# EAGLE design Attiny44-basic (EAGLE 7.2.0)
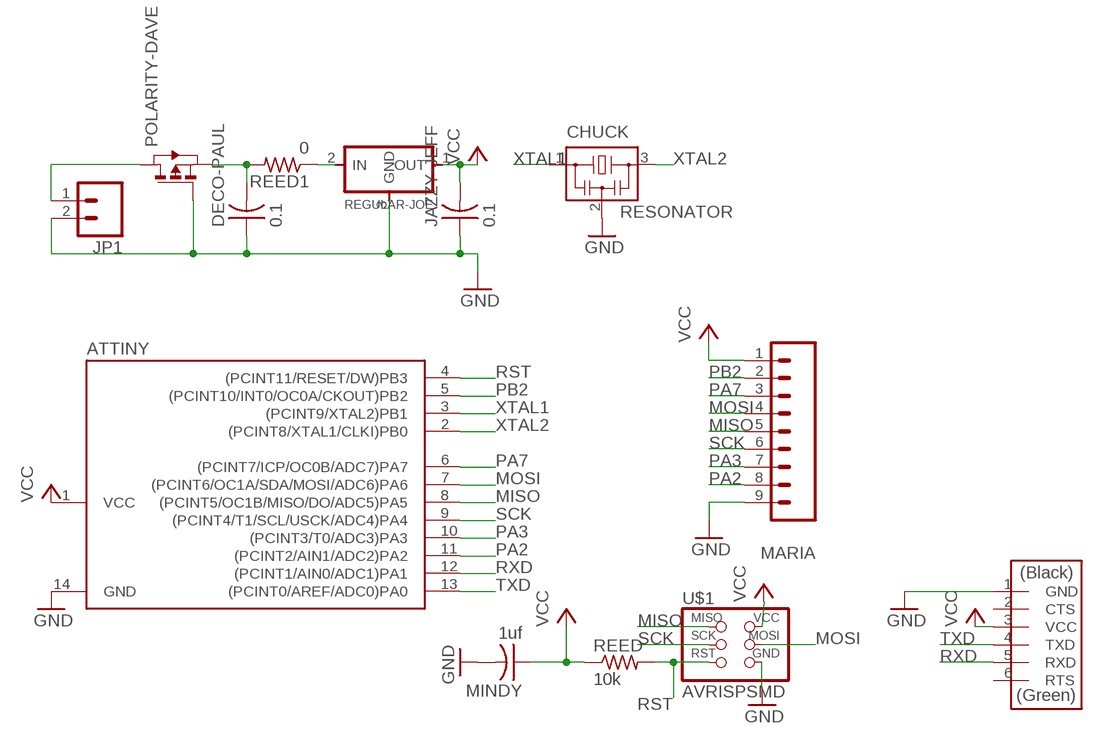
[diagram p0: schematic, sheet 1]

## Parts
ATTINY  ATTINY44-SSU  [SOIC14]
CHUCK  RESONATOR  [EFOBM]
DECO-PAUL  0.1  CAP-US1206  [C1206]
FTDINO  FTDI-SMD-HEADER  [1X06SMD]
JAZZY-JEFF  0.1  CAP-US1206  [C1206]
JP1  M02POLAR_LOCK  [MOLEX-1X2_LOCK]
MARIA  M09LONGPADS  [1X09_LONGPADS]
MINDY  1uf  CAP-US1206  [C1206]
POLARITY-DAVE  PMOSFETSOT23  [SOT-23]
REED  10k  RES-US1206  [R1206]
REED1  0  RES-US1206  [R1206]
REGULAR-JOE  REGULATORSOT23  [SOT23]
U$1  AVRISPSMD  [2X03SMD]

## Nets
GND: ATTINY.14(GND) CHUCK.2 DECO-PAUL.1 FTDINO.1(GND) JAZZY-JEFF.1 JP1.2 MARIA.9 MINDY.2 POLARITY-DAVE.3(G) REGULAR-JOE.3(GND) U$1.6(GND)
MISO: ATTINY.8((PCINT5/OC1B/MISO/DO/ADC5)PA5) MARIA.5 U$1.1(MISO)
MOSI: ATTINY.7((PCINT6/OC1A/SDA/MOSI/ADC6)PA6) MARIA.4 U$1.4(MOSI)
N$1: DECO-PAUL.2 POLARITY-DAVE.2(S) REED1.2
N$3: REED1.1 REGULAR-JOE.2(IN)
N$6: JP1.1 POLARITY-DAVE.1(D)
PA2: ATTINY.11((PCINT2/AIN1/ADC2)PA2) MARIA.8
PA3: ATTINY.10((PCINT3/T0/ADC3)PA3) MARIA.7
PA7: ATTINY.6((PCINT7/ICP/OC0B/ADC7)PA7) MARIA.3
PB2: ATTINY.5((PCINT10/INT0/OC0A/CKOUT)PB2) MARIA.2
RST: ATTINY.4((PCINT11/RESET/DW)PB3) REED.2 U$1.5(RST)
RXD: ATTINY.12((PCINT1/AIN0/ADC1)PA1) FTDINO.5(RXD)
SCK: ATTINY.9((PCINT4/T1/SCL/USCK/ADC4)PA4) MARIA.6 U$1.3(SCK)
TXD: ATTINY.13((PCINT0/AREF/ADC0)PA0) FTDINO.4(TXD)
VCC: ATTINY.1(VCC) FTDINO.3(VCC) JAZZY-JEFF.2 MARIA.1 MINDY.1 REED.1 REGULAR-JOE.1(OUT) U$1.2(VCC)
XTAL1: ATTINY.3((PCINT9/XTAL2)PB1) CHUCK.1
XTAL2: ATTINY.2((PCINT8/XTAL1/CLKI)PB0) CHUCK.3
Unconnected: FTDINO.2(CTS) FTDINO.6(RTS)

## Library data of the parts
ATTINY = 01fab:ATTINY44
CHUCK = 01fab:RESONATOR
DECO-PAUL JAZZY-JEFF MINDY = 01fab:CAP-US
FTDINO = 01fab:FTDI-SMD-HEADER
JP1 = 01_SparkFun:M02: Header 2
MARIA = 01_SparkFun:M09: Header 9 Standard 9-pin 0.1" header. Use with straight break away headers (SKU : PRT-00116), right angle break away headers (PRT-00553), swiss pins (PRT-00743), machine pins (PRT-00117), and female headers (PRT-00115).
POLARITY-DAVE = 01fab:PMOSFET: MOS FET
REED REED1 = 01fab:RES-US: Resistor (US Symbol)
REGULAR-JOE = 01fab:REGULATOR
U$1 = 01fab:AVRISP

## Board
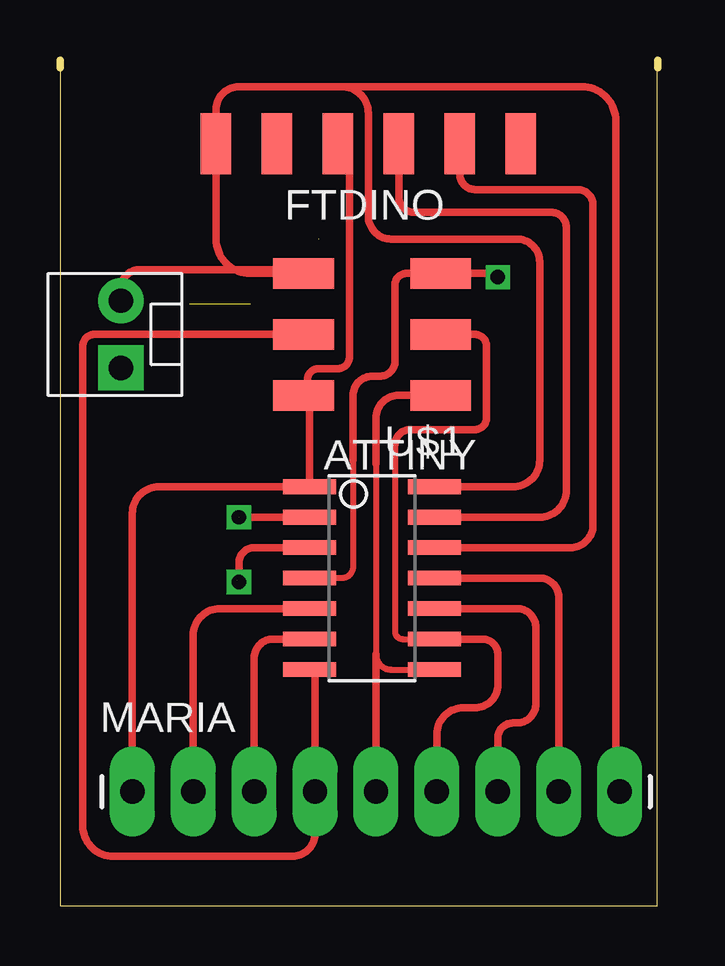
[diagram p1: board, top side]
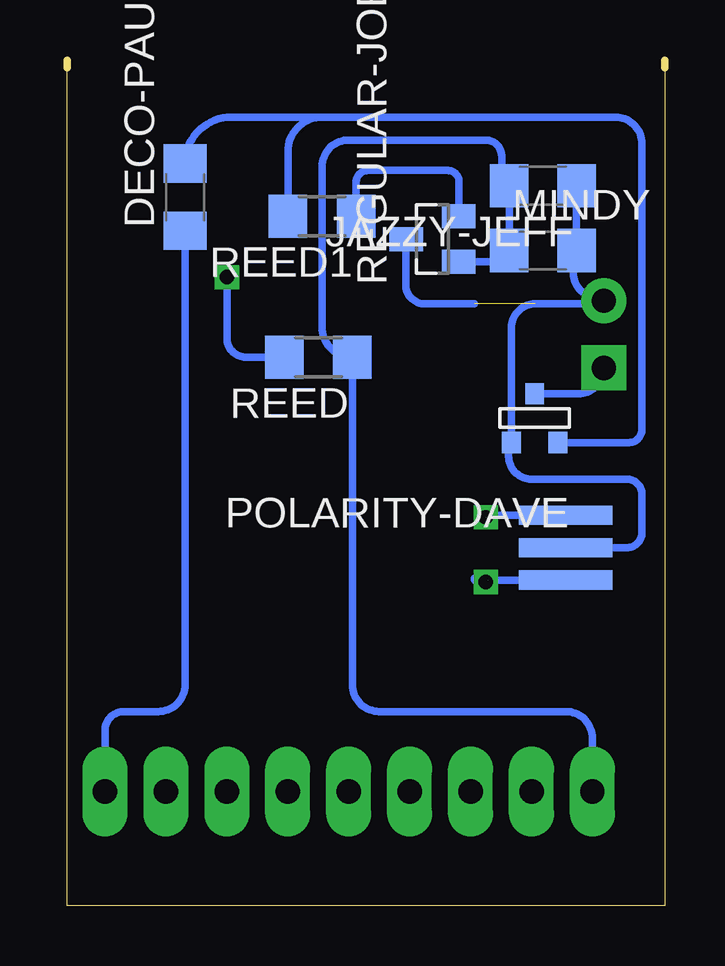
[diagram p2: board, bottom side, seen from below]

Size 24.92 x 35.24 mm. Coordinates in mm from the lower left corner, seen from the top.
Outline: 24.91,35.23 24.91,0 0,0 0,34.93
Outline: 0,35.23 0,34.93
Outline: 24.92,35.24 24.92,34.93
Outline: 0,35.24 0,34.93
Copper layers (1*16): Top 0.035mm / dielectric 1.5mm / Bottom 0.035mm
Design rules "fabmodule": minimum track width 10mil, minimum drill 0.4mm, track to track 0.42mm, track to pad 0.42mm, pad to pad 0.42mm, via to via 0.42mm, smd to smd 0.42mm, copper to edge 40mil, drill to drill 0.8mm, minimum pad ring 10mil, minimum via ring 8mil, stop-mask expansion 4mil, vias tented up to drill 0mil, thermal gap 10mil

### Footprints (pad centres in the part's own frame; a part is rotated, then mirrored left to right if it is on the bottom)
SOIC14 = smd 0.61 x 2.21: 1 -3.81,-2.603; 2 -2.54,-2.603; 3 -1.27,-2.603; 4 0,-2.603; 5 1.27,-2.603; 6 2.54,-2.603; 7 3.81,-2.603; 8 3.81,2.603; 9 2.54,2.603; 10 1.27,2.603; 11 0,2.603; 12 -1.27,2.603; 13 -2.54,2.603; 14 -3.81,2.603
EFOBM = smd 0.8 x 3.9: 1 -1.35,0; 2 0,0; 3 1.35,0
C1206 = smd 1.6 x 1.8: 1 -1.4,0; 2 1.4,0
1X06SMD = smd 2.54 x 1.27: 1 0,6.35; 2 0,3.81; 3 0,1.27; 4 0,-1.27; 5 0,-3.81; 6 0,-6.35
MOLEX-1X2_LOCK = drill 1.016 pad 1.88 square: 1 -0.127,0 | drill 1.016 pad 1.88: 2 2.667,0
1X09_LONGPADS = drill 1.016 pad 1.88 long: 1 0,0; 2 2.54,0; 3 5.08,0; 4 7.62,0; 5 10.16,0; 6 12.7,0; 7 15.24,0; 8 17.78,0; 9 20.32,0
SOT-23 = smd 0.787 x 0.889: 1 0.025,-1.016; 2 -0.94,1.016; 3 0.991,1.016
R1206 = smd 1.6 x 1.803: 1 -1.422,0; 2 1.422,0
SOT23 = smd 1 x 1.4: 1 -0.95,-1.1; 2 0.95,-1.1; 3 0,1.1
2X03SMD = smd 2.54 x 1.27: 1 -2.857,2.54; 2 2.857,2.54; 3 -2.857,0; 4 2.857,0; 5 -2.857,-2.54; 6 2.857,-2.54

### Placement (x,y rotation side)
ATTINY  13.02,13.65 270 top
CHUCK  4.13,14.92 90 bottom
DECO-PAUL  20,29.53 90 bottom
FTDINO  12.86,31.75 90 top
JAZZY-JEFF  5.08,30 180 bottom
JP1  2.54,22.54 90 top
MARIA  3.02,4.76 0 top
MINDY  5.08,27.31 0 bottom
POLARITY-DAVE  5.4,20.32 180 bottom
REED  14.45,22.86 180 bottom
REED1  14.29,28.73 180 bottom
REGULAR-JOE  9.68,27.78 90 bottom
U$1  13.02,23.81 180 top

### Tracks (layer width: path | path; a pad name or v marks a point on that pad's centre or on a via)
GND  (3 unrouted)
  Top 0.305: 9.53,26.35 7.94,26.35 arc-90 6.51,27.78 FTDINO.1 6.51,33.18 arc-90 7.46,34.13 11.75,34.13 | 9.53,26.35 U$1.6 | 11.75,34.13 arc-90 12.86,33.02 12.86,28.73 arc90 13.81,27.78 19.05,27.78 arc-90 20,26.83 20,18.57 arc-90 18.89,17.46 ATTINY.14 | JP1.2 2.54,25.72 arc-90 3.33,26.51 9.37,26.51 arc-90 9.53,26.35 | 11.75,34.13 21.75,34.13 arc-90 23.18,32.7 23.18,4.92 arc90 MARIA.9
  Bottom 0.305: CHUCK.2 1.59,14.92 arc-90 0.95,15.56 0.95,17.14 arc-90 1.59,17.78 5.56,17.78 arc90 6.51,18.73 6.51,19.18 arc90 POLARITY-DAVE.3 6.39,24.09 arc90 5.4,25.08 2.67,25.08 arc-90 JP1.2 arc-90 2.38,25.37 2.83,25.37 arc90 3.81,26.35 3.81,27.18 arc90 MINDY.2 JAZZY-JEFF.1 | 7.94,25.08 10,25.08 arc90 10.8,25.88 10.8,27.77 | DECO-PAUL.1 20,9.21 arc90 21.11,8.1 22.54,8.1 arc-90 23.34,7.3 MARIA.9
MISO
  Top 0.254: 15.46,10 arc-90 ATTINY.8 13.81,9.84 arc-90 13.18,10.48 13.18,18.41
  Top 0.305: U$1.1 14.13,21.27 arc90 13.18,20.32 13.18,18.41 | 13.18,10.48 MARIA.5
MOSI
  Top 0.305: MARIA.4 10.64,9.62 arc90 ATTINY.7 10.48,9.84 | MARIA.4 10.64,9.68 | 10.64,9.68 arc90 10.48,9.84 | 10.48,9.84 arc-90 10.64,9.68 | MARIA.4 10.64,3.02 arc-90 9.68,2.06 2.22,2.06 arc-90 0.95,3.33 0.95,23.34 arc-90 1.43,23.81 U$1.4
N$1
  Bottom 0.305: POLARITY-DAVE.2 1.49,19.3 arc-90 0.95,19.84 0.95,31.75 arc-90 2.06,32.86 14.29,32.86 | 14.29,32.86 18.07,32.86 arc-90 DECO-PAUL.2 | REED1.2 15.71,31.44 arc90 14.29,32.86
N$2  (via drill 0.6)
  other vias: 7.46,16.19
N$3
  Bottom 0.305: REED1.1 12.87,30.16 arc90 12.38,30.64 9.05,30.64 arc90 8.57,30.16 8.57,28.74 arc90 REGULAR-JOE.2
N$4  (via drill 0.6)
  other vias: 7.46,13.49
N$6
  Bottom 0.305: POLARITY-DAVE.1 3.62,21.34 arc-90 JP1.1
PA2
  Top 0.305: ATTINY.11 20,13.65 arc-90 20.8,12.86 MARIA.8
PA3
  Top 0.305: ATTINY.10 19.05,12.38 arc-90 19.84,11.59 19.84,8.41 arc-90 19.05,7.62 18.89,7.62 arc90 18.26,6.98 MARIA.7
PA7
  Top 0.305: MARIA.3 8.1,10.32 arc-90 8.89,11.11 ATTINY.6
PB2
  Top 0.305: MARIA.2 5.56,11.27 arc-90 6.67,12.38 ATTINY.5
RST  (via drill 0.6)
  Top 0.254: 12.22,18.57 12.22,14.13 arc-90 11.75,13.65 ATTINY.4
  Top 0.305: 12.22,18.57 12.22,21.27 arc-90 13.02,22.07 13.33,22.07 arc90 13.97,22.7 13.97,25.88 arc-90 14.45,26.35 U$1.5 | U$1.5 18.41,26.35 | U$1.5 18.1,26.35 arc-90 v18.26,26.19
  Bottom 0.305: 17.46,22.86 arc90 18.26,23.65 | REED.2 17.46,22.86 | 17.46,22.86 arc90 18.26,23.65 | 18.26,23.65 v18.26,26.19 18.26,26.35
RXD
  Top 0.305: FTDINO.5 16.67,30.48 arc90 17.3,29.85 21.59,29.85 arc-90 22.23,29.21 22.23,15.87 arc-90 21.27,14.92 ATTINY.12
SCK
  Top 0.254: 13.97,19.21 13.97,11.43 arc90 14.29,11.11 ATTINY.9
  Top 0.305: U$1.3 17.3,23.81 arc-90 17.78,23.34 17.78,20.32 arc-90 17.3,19.84 14.61,19.84 arc90 13.97,19.21 | MARIA.6 15.72,7.14 arc-90 16.83,8.25 17.3,8.25 arc90 18.26,9.21 18.26,10.48 arc90 17.62,11.11 ATTINY.9
TXD
  Top 0.305: ATTINY.13 20,16.19 arc90 21.11,17.3 21.11,28.26 arc90 20.48,28.89 14.76,28.89 arc-90 14.13,29.53 FTDINO.4
VCC
  Top 0.305: FTDINO.3 11.59,31.11 arc90 12.06,30.64 12.06,22.86 arc-90 11.59,22.38 10.8,22.38 arc90 10.32,21.91 10.32,21.43 arc90 10.48,21.27 U$1.2 10.41,21.27 ATTINY.1 4.13,17.46 arc90 3.02,16.35 MARIA.1
  Bottom 0.305: REGULAR-JOE.1 6.95,26.83 arc-90 MINDY.1 JAZZY-JEFF.2 arc-90 6.8,30.32 6.8,31.25 arc-90 7.46,31.91 13.18,31.91 arc-90 14.29,30.8 14.29,24.12 arc-90 REED.1 13.02,9.21 arc-90 11.91,8.1 4.13,8.1 arc90 3.02,6.98 MARIA.1
XTAL1  (1 unrouted)
  Top 0.305: ATTINY.3 8.1,14.92 arc90 7.46,14.29 7.46,13.65 arc-90 7.38,13.57
  Bottom 0.305: CHUCK.1 7.38,13.57 arc-90 7.46,13.49 7.78,13.49 arc90 7.94,13.65
XTAL2  (1 unrouted)
  Top 0.305: ATTINY.2 7.46,16.19
  Bottom 0.305: CHUCK.3 7.38,16.27 arc-90 7.46,16.19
